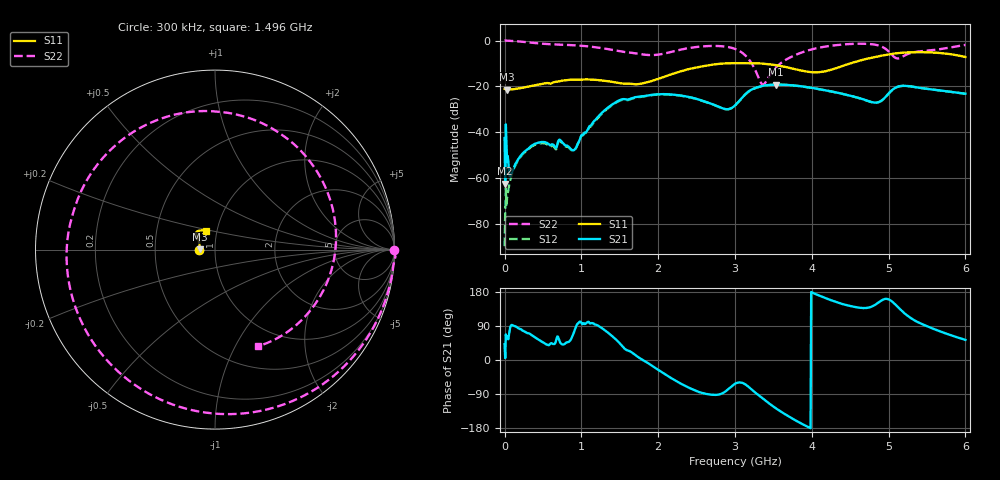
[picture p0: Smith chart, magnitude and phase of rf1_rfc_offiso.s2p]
!Agilent Technologies,M9375A,MY55441453,A.02.50.04
!Agilent M9375A: A.02.50.04
!Date: Monday, December 12, 2016 11:32:16
!Correction: S11(Full 2 Port(1,2))
!S21(Full 2 Port(1,2))
!S12(Full 2 Port(1,2))
!S22(Full 2 Port(1,2))
!S2P File: Measurements: S11, S21, S12, S22:
# Hz S  dB  R 50
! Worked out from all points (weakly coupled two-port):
!   751 points, 300 kHz to 6 GHz, reference 50 ohm
!   highest |S21| = -19.23 dB at 3.536 GHz (marker M1); lowest = -62.5 dB at 8.3 MHz (marker M2)
!   lowest |S11| = -21.4 dB at 32.3 MHz (marker M3), VSWR 1.19, Z = 42.1 + j0.232 ohm
!   |S11| at or under -10 dB: start of sweep to 2.861 GHz; 3.336 GHz to 4.498 GHz (1.162 GHz wide, 29.7 % of centre)
!   |S22| runs from -19.2 to 0.1 dB; largest |S21 - S12| = 0.014
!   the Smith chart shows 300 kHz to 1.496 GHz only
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300000  -21.07 -177.1  -42.55 41.6  -89.78 66.9  -0.03 -0.2
8299600  -21.17 179.8  -62.53 4.9  -75.34 94.3  0.05 -2.2
3.22984e7  -21.37 178.2  -52.86 62.1  -68.76 95.7  -0.04 -9.6
8.0296e7  -21.32 172.8  -58.93 89.9  -60.15 99.5  -0.13 -23.4
2.882856e8  -20.26 155.6  -47.77 72.0  -48.14 71.6  -0.71 -84.2
5.60272e8  -18.55 141.3  -44.84 39.9  -45.52 39.6  -1.53 -161.4
7.522624e8  -17.48 140.6  -44.43 41.0  -44.85 42.5  -1.82 150.0
1.00025e9  -17.06 136.0  -41.37 98.1  -41.56 97.8  -2.29 88.9
1.272236e9  -17.45 127.8  -31.36 83.4  -31.73 84.0  -3.33 8.6
1.528224e9  -18.74 112.9  -25.67 37.7  -25.89 38.7  -4.80 -76.3
1.776211e9  -18.84 85.2  -24.39 2.8  -24.56 4.0  -5.97 -155.9
2.0002e9  -16.75 58.8  -23.45 -26.0  -23.56 -25.0  -6.14 128.9
2.552172e9  -11.40 34.9  -26.03 -85.8  -26.13 -85.2  -2.61 12.4
3.00015e9  -9.85 33.8  -28.32 -62.7  -28.41 -62.7  -3.64 -61.2
3.232138e9  -9.88 34.9  -21.15 -80.6  -21.24 -80.2  -10.81 -137.6
3.368132e9  -10.09 33.5  -19.71 -102.8  -19.77 -102.3  -19.24 108.2
3.536123e9  -10.75 29.7  -19.23 -128.0  -19.27 -127.4  -11.59 -1.2
4.0001e9  -13.83 -6.8  -20.66 178.6  -20.68 178.8  -3.84 -99.7
4.648068e9  -8.50 -61.6  -25.41 137.4  -25.45 137.5  -1.38 -147.1
5.00005e9  -6.05 -62.6  -23.12 160.1  -23.15 160.2  -4.71 -178.3
5.280036e9  -5.12 -60.9  -19.96 111.9  -19.97 112.1  -5.52 -164.1
6e9  -7.17 -55.3  -23.21 53.1  -23.23 53.2  -1.90 100.5
